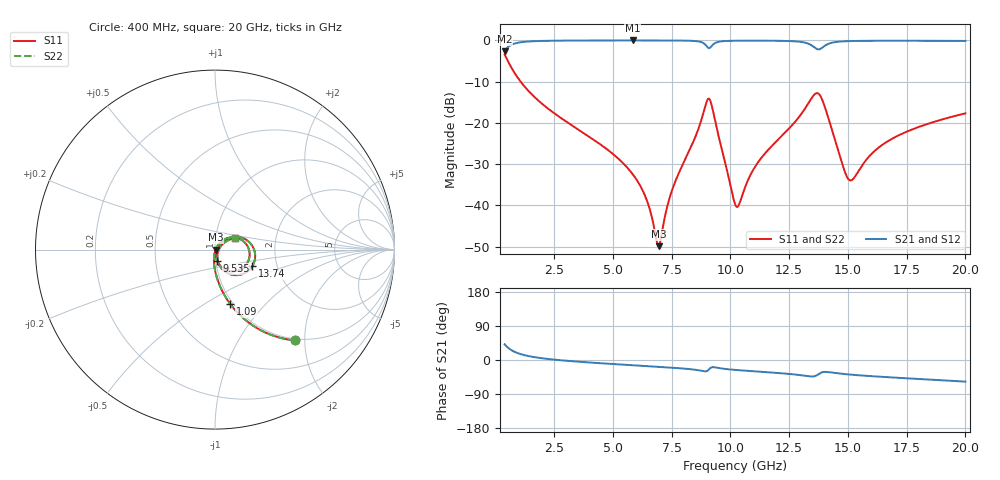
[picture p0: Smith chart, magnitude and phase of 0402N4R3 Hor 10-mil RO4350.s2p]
# GHz S MA R 50
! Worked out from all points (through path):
!   1960 points, 400 MHz to 20 GHz, reference 50 ohm
!   highest |S21| = -0.03 dB at 5.853 GHz (marker M1); lowest = -2.6 dB at 400 MHz (marker M2)
!   group delay of S21, straight-line fit = 9.53 ps
!   lowest |S11| = -49.9 dB at 6.953 GHz (marker M3), VSWR 1.01, Z = 50.3 - j0.104 ohm
!   |S11| at or under -10 dB: 1.079 GHz to end of sweep
!   |S22| runs from -49.9 to -3.4 dB; largest |S21 - S12| = 0
!   S11 on the Smith chart (normalised r, x): 400 MHz: 0.97, -1.80; 1.09 GHz: 0.97, -0.65; 9.535 GHz: 1.02, -0.13; 13.74 GHz: 1.49, -0.29; 20 GHz: 1.24, +0.17
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0.4  0.6745 -48.6  0.738 41.4  0.738 41.4  0.6745 -48.6
0.7101582  0.4556 -64.7  0.8896 25.3  0.8896 25.3  0.4556 -64.7
1.090352  0.3133 -74.4  0.9488 15.4  0.9488 15.4  0.3133 -74.4
3.671669  0.07814 -93.8  0.9951 -5.1  0.9951 -5.1  0.07814 -93.8
5.852782  0.02372 -98.0  0.997 -13.8  0.997 -13.8  0.02372 -98.0
6.443083  0.01161 -92.4  0.9969 -16.1  0.9969 -16.1  0.01161 -92.4
6.943338  0.003192 -23.1  0.9965 -18.0  0.9965 -18.0  0.003192 -23.1
6.953344  0.003192 -18.9  0.9965 -18.0  0.9965 -18.0  0.003192 -18.9
7.523635  0.01526 53.7  0.9954 -20.3  0.9954 -20.3  0.01526 53.7
8.55416  0.07215 48.6  0.9781 -26.1  0.9781 -26.1  0.07215 48.6
9.0244  0.1887 0.4  0.8302 -28.5  0.8302 -28.5  0.1887 0.4
9.184482  0.1729 -42.5  0.8379 -19.9  0.8379 -19.9  0.1729 -42.5
9.534661  0.06301 -79.6  0.9649 -21.5  0.9649 -21.5  0.06301 -79.6
10.205  0.01028 -38.0  0.9895 -26.1  0.9895 -26.1  0.01028 -38.0
10.36508  0.01011 1.0  0.9906 -26.9  0.9906 -26.9  0.01011 1.0
11.21552  0.03429 46.8  0.9916 -30.7  0.9916 -30.7  0.03429 46.8
13.46667  0.2008 9.8  0.8664 -43.5  0.8664 -43.5  0.2008 9.8
13.7368  0.2273 -24.2  0.7772 -38.0  0.7772 -38.0  0.2273 -24.2
14.21705  0.1037 -71.8  0.9172 -32.3  0.9172 -32.3  0.1037 -71.8
15.06748  0.02016 -26.7  0.9796 -38.4  0.9796 -38.4  0.02016 -26.7
16.73834  0.06073 36.3  0.9889 -45.5  0.9889 -45.5  0.06073 36.3
20  0.1304 30.1  0.9841 -57.0  0.9841 -57.0  0.1304 30.1
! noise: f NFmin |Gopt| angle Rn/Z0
0.4  0.00106  0.7538  3.186  0.0008685
2.571  0.004931  0.6712  7.297  0.002875
4.752  0.008136  0.6401  12.64  0.00422
6.933  0.01223  0.6509  17.97  0.006502
9.104  0.119  0.9451  23.48  0.4655
11.29  0.02357  0.7029  28.8  0.01462
13.47  0.108  0.9143  34.23  0.2535
15.64  0.03585  0.733  39.4  0.02382
17.82  0.02886  0.6474  44.11  0.01344
20  0.02892  0.6196  48.67  0.0119
